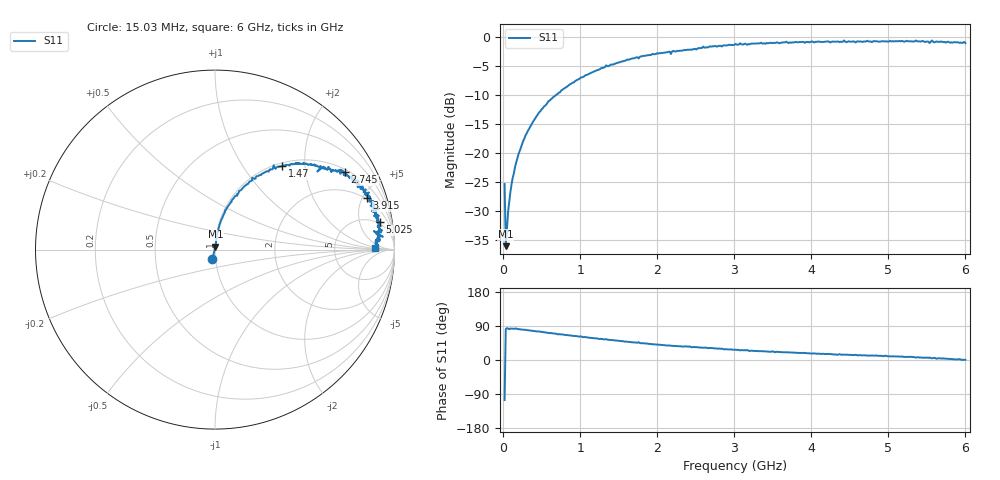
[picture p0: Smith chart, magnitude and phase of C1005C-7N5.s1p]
!	Network	Analyzer	HP8753E.07.74:	Oct	30	2002	Serial	No.	JP38451487
!	Hewlett-Packard
!	7	Sep	2009	8:34:30
!	Frequency	S11
#	HZ	S	RI	R	50
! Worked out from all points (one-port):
!   400 points, 15.03 MHz to 6 GHz, reference 50 ohm
!   lowest |S11| = -36.0 dB at 30.03 MHz (marker M1), VSWR 1.03, Z = 50.2 + j1.58 ohm
!   |S11| at or under -10 dB: start of sweep to 678.9 MHz
!   S11 on the Smith chart (normalised r, x): 15.03 MHz: 0.97, -0.10; 1.47 GHz: 1.05, +1.54; 2.745 GHz: 1.11, +3.28; 3.915 GHz: 1.89, +5.43; 5.025 GHz: 4, +10; 6 GHz: 17, +1
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1.502992e7  -0.0148 -0.0524
3.002985e7  0.0023 0.0157
6.00297e7  0.00376 0.031
1.050295e8  0.00673 0.0536
1.650292e8  0.00944 0.0828
2.400288e8  0.0201 0.118
4.650277e8  0.0561 0.219
7.650262e8  0.134 0.326
1.335023e9  0.327 0.47
1.470023e9  0.376 0.467
1.515022e9  0.391 0.467
2.265019e9  0.613 0.457
2.745016e9  0.723 0.431
3.015015e9  0.779 0.399
3.195014e9  0.796 0.347
3.765011e9  0.847 0.302
3.91501e9  0.847 0.287
4.00501e9  0.881 0.27
4.515007e9  0.889 0.215
5.025005e9  0.918 0.152
5.265004e9  0.915 0.128
5.445003e9  0.925 0.0951
5.535002e9  0.885 0.103
5.565002e9  0.935 0.0719
5.595002e9  0.898 0.0909
5.625002e9  0.919 0.0526
5.655002e9  0.911 0.0757
6e9  0.891 0.00769
